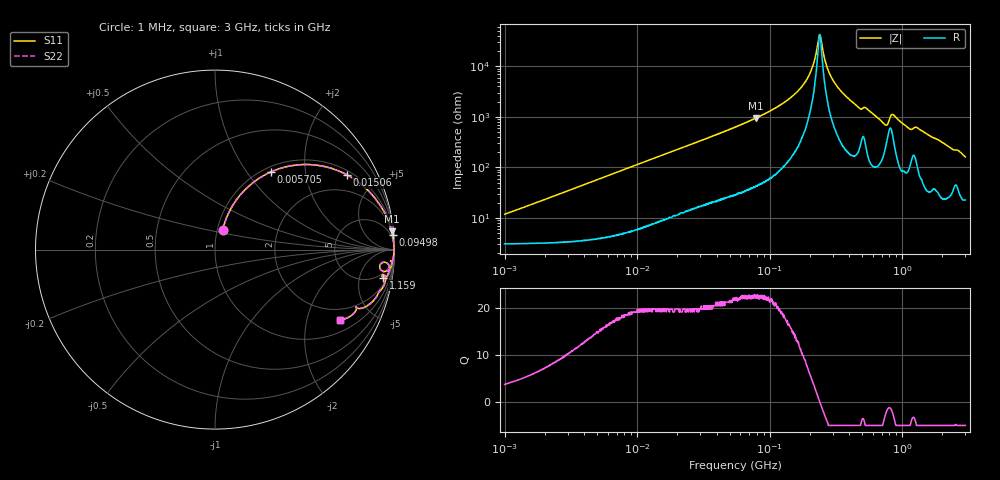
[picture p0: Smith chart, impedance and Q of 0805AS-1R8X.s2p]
!s-Parameter Generated by FASTRON Sdn. Bhd.
!FASTRON P/N : 0805AS-1R8X
!Keysight Technologies: E4991B_MY54100416_A.01.15
!Date: Mon Jun 15 12:57:15 2026
!Version  :Rev01  Mon Jun 15 12:57:15 2026
!Data & Calibration Information:
!Freq  S11  S21  S12  S22
!PortZ  Port1:50+j0  Port2:50+j0
!When reading reference impedance value at option line is always used.
! Remarks : This data is being provided solely for informational purposes.
# Hz S dB R 50
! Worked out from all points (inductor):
!   1601 points, 1 MHz to 3 GHz, reference 50 ohm
!   read as one part in series: L = 1.83 uH near 1.041 MHz
!   highest Q = 22.5 at 79.32 MHz (marker M1), where L = 1.92 uH
!   self-resonance near 238.5 MHz
!   S11 on the Smith chart (normalised r, x): 1 MHz: 1.06, +0.23; 5.705 MHz: 1.08, +1.31; 15.06 MHz: 1.17, +3.41; 94.98 MHz: 2, +24; 1.159 GHz: 3, -11; 3 GHz: 1.46, -3.18
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1000000  -18.80 68.6  -0.32 -6.4  -0.32 -6.4  -18.80 68.6
3804036  -8.20 62.5  -1.01 -22.8  -1.01 -22.8  -8.20 62.5
5705239  -5.48 54.3  -1.79 -32.1  -1.79 -32.1  -5.48 54.3
1.447069e7  -1.57 30.6  -5.86 -56.5  -5.86 -56.5  -1.57 30.6
1.506173e7  -1.47 29.6  -6.11 -57.4  -6.11 -57.4  -1.47 29.6
5.504702e7  -0.17 9.0  -16.10 -78.4  -16.10 -78.4  -0.17 9.0
7.931905e7  -0.09 5.9  -19.70 -81.5  -19.70 -81.5  -0.09 5.9
9.497575e7  -0.06 4.7  -21.70 -82.7  -21.70 -82.7  -0.06 4.7
1.582265e8  -0.03 1.9  -29.50 -83.9  -29.50 -83.9  -0.03 1.9
2.083556e8  -0.02 0.6  -39.10 -77.4  -39.10 -77.4  -0.02 0.6
2.396927e8  -0.02 -0.0  -52.50 4.3  -52.50 4.3  -0.02 -0.0
2.785165e8  -0.02 -0.7  -38.10 78.1  -38.10 78.1  -0.02 -0.7
3.402349e8  -0.03 -1.7  -30.60 82.7  -30.60 82.7  -0.03 -1.7
4.686663e8  -0.09 -3.7  -23.80 78.5  -23.80 78.5  -0.09 -3.7
5.364635e8  -0.11 -3.8  -23.50 77.4  -23.50 77.4  -0.11 -3.8
7.316083e8  -0.38 -7.3  -17.60 67.3  -17.60 67.3  -0.38 -7.3
7.925923e8  -0.68 -5.1  -18.90 46.3  -18.90 46.3  -0.68 -5.1
8.543737e8  -0.30 -4.7  -21.20 65.0  -21.20 65.0  -0.30 -4.7
1.159346e9  -0.44 -9.4  -15.50 68.3  -15.50 68.3  -0.44 -9.4
1.287806e9  -0.36 -8.8  -16.20 70.4  -16.20 70.4  -0.36 -8.8
1.960646e9  -0.58 -16.6  -10.80 68.9  -10.80 68.9  -0.58 -16.6
3e9  -1.94 -29.5  -6.07 52.4  -6.07 52.4  -1.94 -29.5
